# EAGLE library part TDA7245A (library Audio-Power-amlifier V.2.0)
The TDA7245A is a monolithic integrated circuit in 9+9 POWERDIP package, intended for use as low frequency power amplifier in a wide range of applications in radio and TV sets.
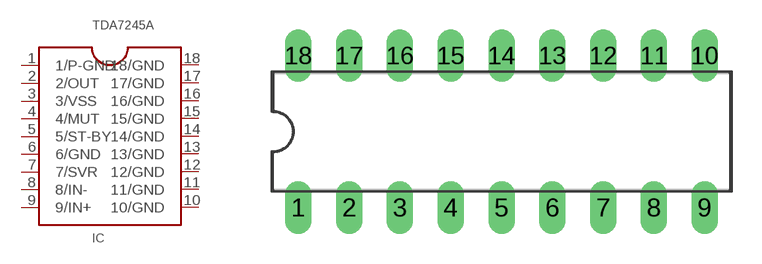
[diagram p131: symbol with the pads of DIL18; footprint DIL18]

Designator prefix IC

## TDA7245A  [DIL18]
1  1/P-GND  pwr
2  2/OUT  out
3  3/VSS  pwr
4  4/MUT  in
5  5/ST-BY  in
6  6/GND  pwr
7  7/SVR
8  8/IN-  in
9  9/IN+  in
10  10/GND  pwr
11  11/GND  pwr
12  12/GND  pwr
13  13/GND  pwr
14  14/GND  pwr
15  15/GND  pwr
16  16/GND  pwr
17  17/GND  pwr
18  18/GND  pwr

## Footprint DIL18 (pad centres in mm)
Dual In Line Package
drill 0.813 long: 1 -10.16,-3.81; 2 -7.62,-3.81; 3 -5.08,-3.81; 4 -2.54,-3.81; 5 0,-3.81; 6 2.54,-3.81; 7 5.08,-3.81; 8 7.62,-3.81; 9 10.16,-3.81; 10 10.16,3.81; 11 7.62,3.81; 12 5.08,3.81; 13 2.54,3.81; 14 0,3.81; 15 -2.54,3.81; 16 -5.08,3.81; 17 -7.62,3.81; 18 -10.16,3.81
